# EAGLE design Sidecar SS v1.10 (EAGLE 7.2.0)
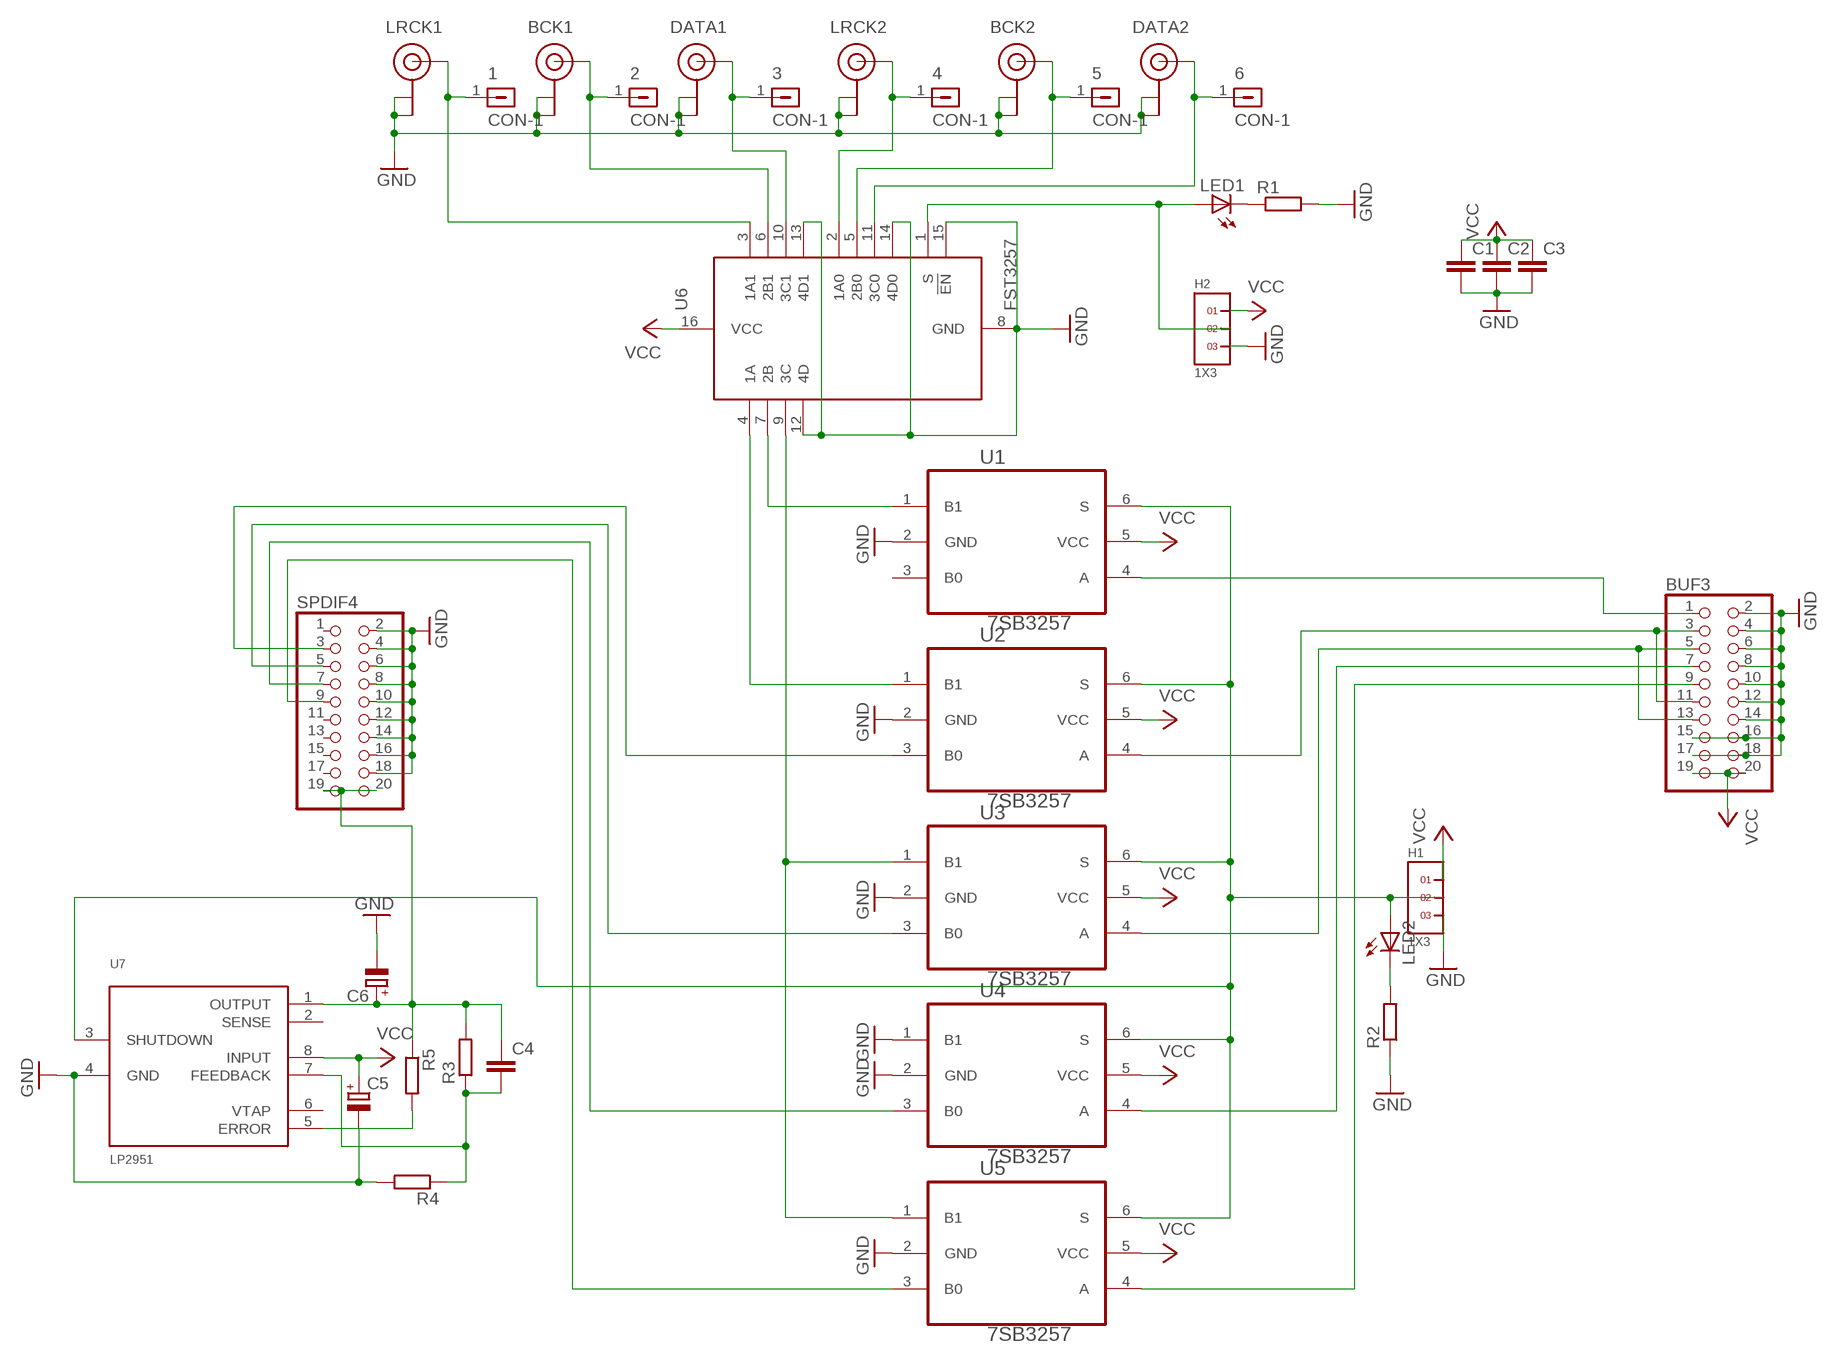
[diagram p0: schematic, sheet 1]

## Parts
1  CON-1  [CON-1]
2  CON-1  [CON-1]
3  CON-1  [CON-1]
4  CON-1  [CON-1]
5  CON-1  [CON-1]
6  CON-1  [CON-1]
BCK1  U.FL  [U.FL]
BCK2  U.FL  [U.FL]
BUF3  PINHD-2X10  [2X10]
C1  C-EUC0805  [C0805]
C2  C-EUC0805  [C0805]
C3  C-EUC0805  [C0805]
C4  C-EUC1206  [C1206]
C5  CPOL-EUCT3216  [CT3216]
C6  CPOL-EUCT3216  [CT3216]
DATA1  U.FL  [U.FL]
DATA2  U.FL  [U.FL]
H1  1X3  [1X3]
H2  1X3  [1X3]
LED1  LED_E  [LED_1206]
LED2  LED_E  [LED_1206]
LRCK1  U.FL  [U.FL]
LRCK2  U.FL  [U.FL]
R1  R-EU_R1206  [R1206]
R2  R-EU_R1206  [R1206]
R3  R-EU_R1206  [R1206]
R4  R-EU_R1206  [R1206]
R5  R-EU_R1206  [R1206]
SPDIF4  PINHD-2X10  [2X10]
U1  7SB3257  [TSOP-6]
U2  7SB3257  [TSOP-6]
U3  7SB3257  [TSOP-6]
U4  7SB3257  [TSOP-6]
U5  7SB3257  [TSOP-6]
U6  FST3257  [TSSOP16]
U7  LP2951  [SOIC-8]

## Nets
GND: BCK1.P$1(GND) BCK1.P$2(GND) BCK2.P$1(GND) BCK2.P$2(GND) BUF3.2 BUF3.4 BUF3.6 BUF3.8 BUF3.10 BUF3.12 BUF3.14 BUF3.15 BUF3.16 BUF3.17 BUF3.18 C1.2 C2.2 C3.2 C5.- C6.- DATA1.P$1(GND) DATA1.P$2(GND) DATA2.P$1(GND) DATA2.P$2(GND) H1.3 H2.3 LRCK1.P$1(GND) LRCK1.P$2(GND) LRCK2.P$1(GND) LRCK2.P$2(GND) R1.2 R2.1 R4.2 SPDIF4.2 SPDIF4.4 SPDIF4.6 SPDIF4.8 SPDIF4.10 SPDIF4.12 SPDIF4.14 SPDIF4.16 SPDIF4.18 U1.2(GND) U2.2(GND) U3.2(GND) U4.1(B1) U4.2(GND) U5.2(GND) U6.8(GND) U6.12(4D) U6.13(4D1) U6.14(4D0) U6.15(!EN) U7.4(GND)
N$1: C4.2 R3.1 R4.1 U7.7(FEEDBACK)
N$2: U1.1(B1) U6.7(2B)
N$3: SPDIF4.3 U2.3(B0)
N$4: BUF3.5 BUF3.13 U3.4(A)
N$5: BUF3.3 BUF3.11 U2.4(A)
N$6: BUF3.1 U1.4(A)
N$7: SPDIF4.5 U3.3(B0)
N$8: SPDIF4.7 U4.3(B0)
N$9: BUF3.7 U4.4(A)
N$10: BUF3.9 U5.4(A)
N$11: SPDIF4.9 U5.3(B0)
N$12: H1.2 LED2.A U1.6(S) U2.6(S) U3.6(S) U4.6(S) U5.6(S) U7.3(SHUTDOWN)
N$14: LED1.C R1.1
N$15: U2.1(B1) U6.4(1A)
N$16: U3.1(B1) U5.1(B1) U6.9(3C)
N$17: 1.1 LRCK1.P$3(SIGNAL) U6.3(1A1)
N$18: 2.1 BCK1.P$3(SIGNAL) U6.6(2B1)
N$19: 3.1 DATA1.P$3(SIGNAL) U6.10(3C1)
N$20: 4.1 LRCK2.P$3(SIGNAL) U6.2(1A0)
N$21: 5.1 BCK2.P$3(SIGNAL) U6.5(2B0)
N$22: 6.1 DATA2.P$3(SIGNAL) U6.11(3C0)
N$23: LED2.C R2.2
N$25: C4.1 C6.+ R3.2 R5.1 SPDIF4.19 SPDIF4.20 U7.1(OUTPUT)
N$27: R5.2 U7.5(ERROR)
N$29: H2.2 LED1.A U6.1(S)
VCC: BUF3.19 BUF3.20 C1.1 C2.1 C3.1 C5.+ H1.1 H2.1 U1.5(VCC) U2.5(VCC) U3.5(VCC) U4.5(VCC) U5.5(VCC) U6.16(VCC) U7.8(INPUT)
Unconnected: SPDIF4.1 SPDIF4.11 SPDIF4.13 SPDIF4.15 SPDIF4.17 U1.3(B0) U7.2(SENSE) U7.6(VTAP)

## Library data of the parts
1-6 = Dimdim:CON-1
BCK1 BCK2 DATA1 DATA2 LRCK1 LRCK2 = Dimdim:U.FL
BUF3 SPDIF4 = SparkFun-Connectors:PINHD-2X10: PIN HEADER
C1-C4 = rcl:C-EU: CAPACITOR, European symbol
C5 C6 = rcl:CPOL-EU: POLARIZED CAPACITOR, European symbol
H1 H2 = headers(.1in):1X3
LED1 LED2 = eagle-ltspice:LED_E: LED; SPICEMODEL: NONE; SPICEPREFIX: D; SPICETYPE: diode
R1-R5 = rcl:R-EU_: RESISTOR, European symbol
U1-U5 = Dimdim:7SB3257
U6 = Dimdim:FST3257
U7 = Dimdim:LP2951

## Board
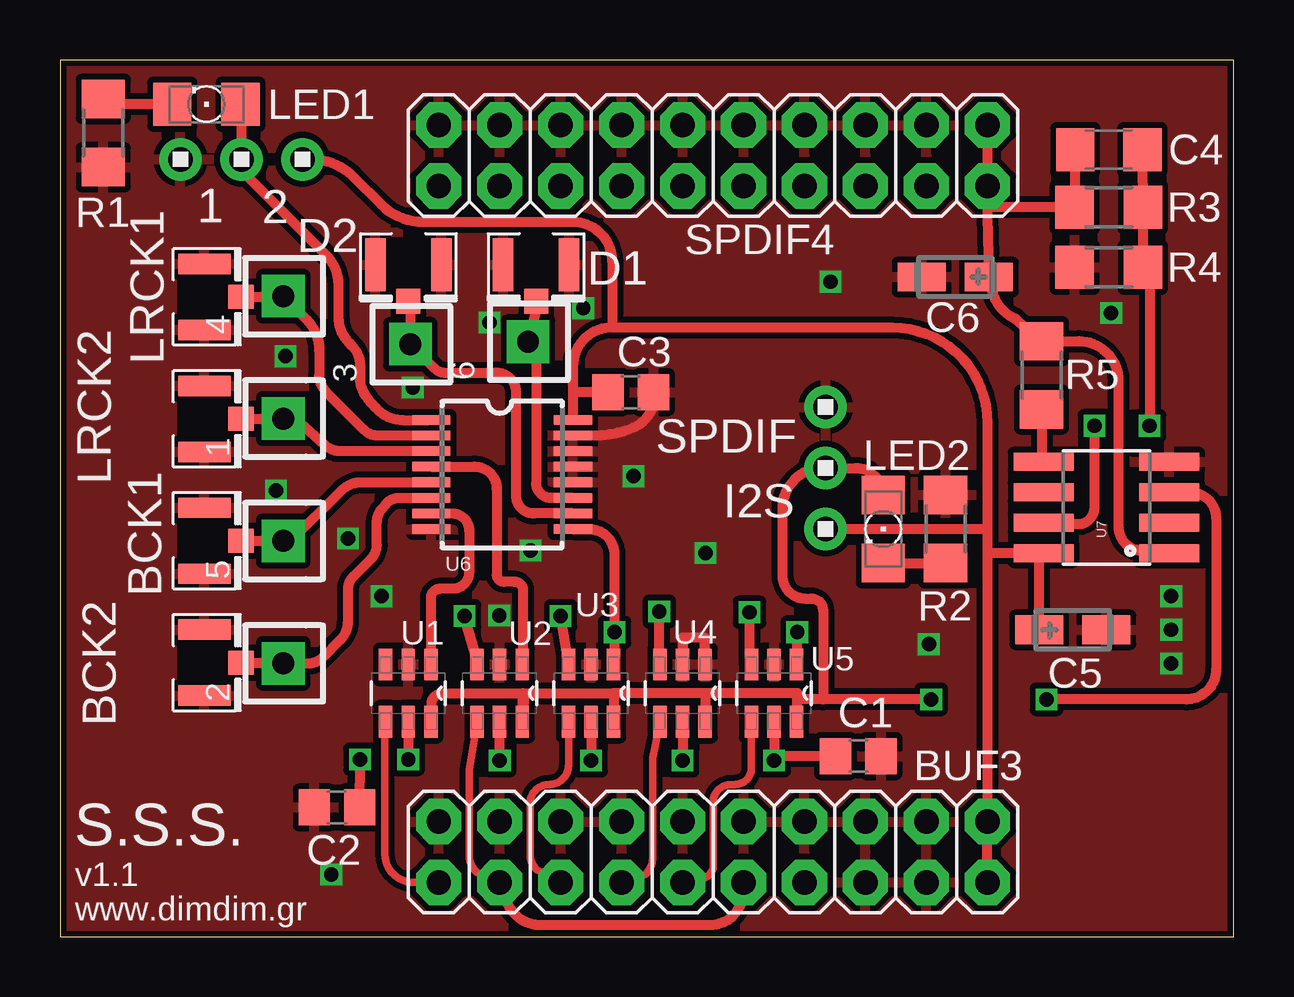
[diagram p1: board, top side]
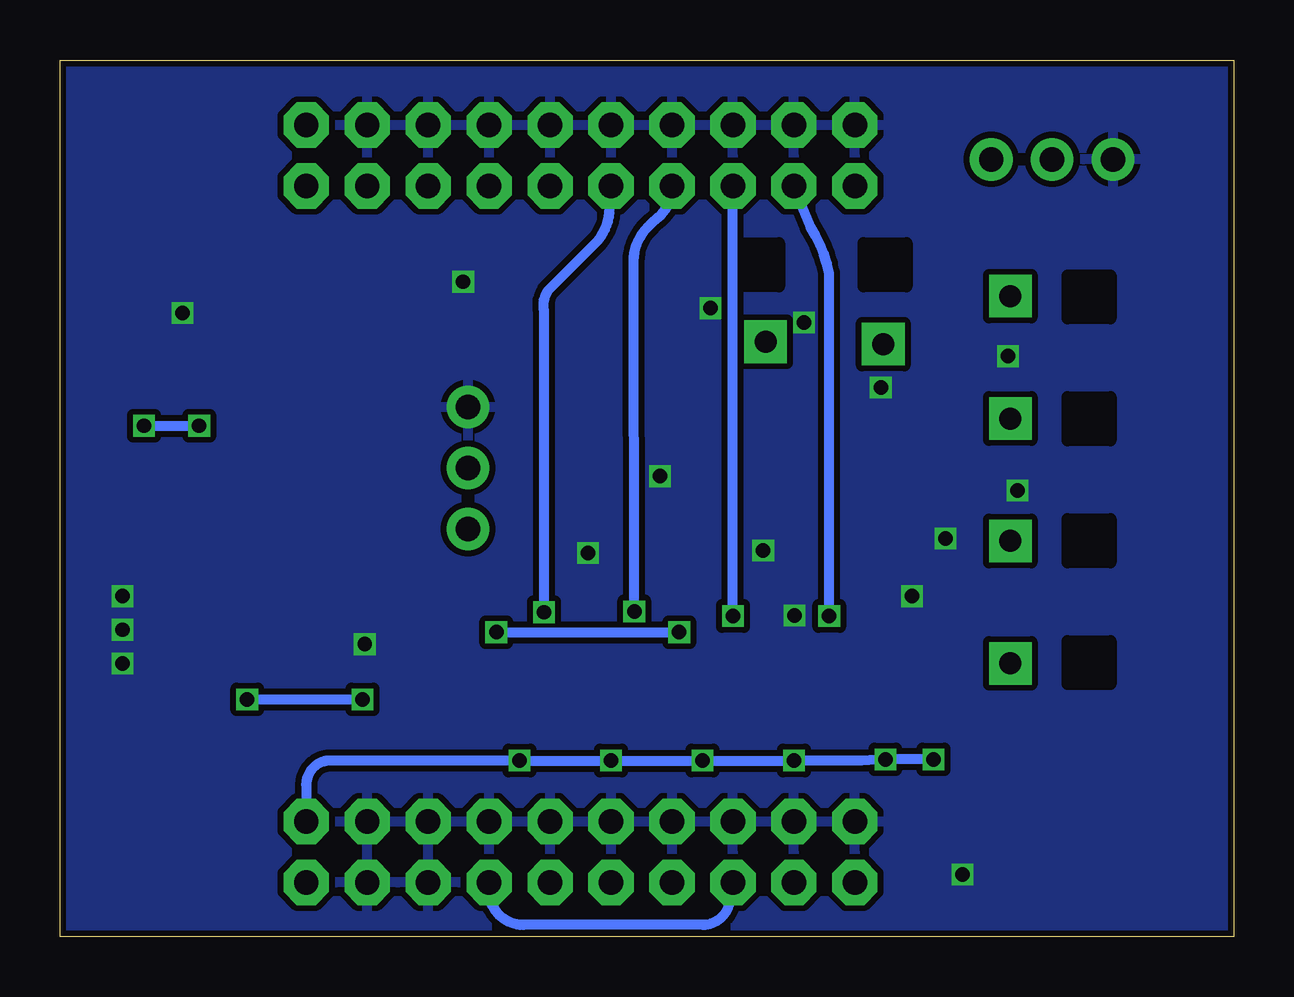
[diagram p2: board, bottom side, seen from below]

Size 48.9 x 36.54 mm. Coordinates in mm from the lower left corner, seen from the top.
Outline: 0,0 48.9,0 48.9,36.54 0,36.54 0,0
Copper layers (1*16): Top 0.035mm / dielectric 1.5mm / Bottom 0.035mm
Design rules "SeeedStudio_2layer_DRU_no_angle_20140221": minimum track width 6mil, minimum drill 12mil, track to track 6mil, track to pad 6mil, pad to pad 6mil, via to via 6mil, smd to smd 0mil, copper to edge 10mil, drill to drill 10mil, minimum pad ring 10mil, minimum via ring 6mil, stop-mask expansion 2mil, vias tented up to drill 100mil, thermal gap 10mil

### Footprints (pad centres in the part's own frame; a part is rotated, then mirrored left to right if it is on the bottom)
CON-1 = drill 0.914 pad 1.778 square: 1 0,0
U.FL = smd 2.2 x 0.85: P$1 0,1.375; P$2 0,-1.375 | smd 1.05 x 1: P$3 1.525,0
2X10 = drill 1.016 pad 1.88 octagon: 1 -11.43,-1.27; 2 -11.43,1.27; 3 -8.89,-1.27; 4 -8.89,1.27; 5 -6.35,-1.27; 6 -6.35,1.27; 7 -3.81,-1.27; 8 -3.81,1.27; 9 -1.27,-1.27; 10 -1.27,1.27; 11 1.27,-1.27; 12 1.27,1.27; 13 3.81,-1.27; 14 3.81,1.27; 15 6.35,-1.27; 16 6.35,1.27; 17 8.89,-1.27; 18 8.89,1.27; 19 11.43,-1.27; 20 11.43,1.27
C0805 = smd 1.3 x 1.5: 1 -0.95,0; 2 0.95,0
C1206 = smd 1.6 x 1.8: 1 -1.4,0; 2 1.4,0
CT3216 = smd 2 x 1.2: + -1.4,0; - 1.4,0
1X3 = drill 1.016 pad 1.778: 1 0,0; 2 2.54,0; 3 5.08,0
LED_1206 = smd 1.6 x 1.803: A -1.422,0; C 1.422,0
R1206 = smd 1.6 x 1.803: 1 -1.422,0; 2 1.422,0
TSOP-6 = smd 1.321 x 0.559: 1 -1.194,2.21; 2 -1.194,1.27; 3 -1.194,0.33; 4 1.194,0.33; 5 1.194,1.27; 6 1.194,2.21
TSSOP16 = smd 0.4 x 1.6: 1 -2.225,-2.85; 2 -1.575,-2.85; 3 -0.925,-2.85; 4 -0.275,-2.85; 5 0.375,-2.85; 6 1.025,-2.85; 7 1.675,-2.85; 8 2.325,-2.85; 9 2.325,3.05; 10 1.675,3.05; 11 1.025,3.05; 12 0.375,3.05; 13 -0.275,3.05; 14 -0.925,3.05; 15 -1.575,3.05; 16 -2.225,3.05
SOIC-8 = smd 0.75 x 2.5: 1 -1.905,-2.616; 2 -0.635,-2.616; 3 0.635,-2.616; 4 1.905,-2.616; 5 1.905,2.616; 6 0.635,2.616; 7 -0.635,2.616; 8 -1.905,2.616

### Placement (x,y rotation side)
1  9.3,21.6 0 top
2  9.3,11.4 0 top
3  14.6,24.7 0 top
4  9.3,26.7 0 top
5  9.3,16.5 0 top
6  19.5,24.8 0 top
BCK1  6.02,11.43 0 top
BCK2  6.02,16.51 0 top
BUF3  27.21,3.54 0 top
C1  33.26,7.54 0 top
C2  11.54,5.4 180 top
C3  23.78,22.7 0 top
C4  43.7,32.8 0 top
C5  42.2,12.8 0 top
C6  37.3,27.5 180 top
DATA1  14.52,28.01 270 top
DATA2  19.84,28.01 270 top
H1  31.9,17 90 top
H2  10.1,32.4 180 top
LED1  6.1,34.7 180 top
LED2  34.3,17 270 top
LRCK1  6.02,21.59 0 top
LRCK2  6.02,26.67 0 top
R1  1.8,33.5 270 top
R2  36.9,17 270 top
R3  43.7,30.4 180 top
R4  43.7,27.9 180 top
R5  40.9,23.4 270 top
SPDIF4  27.21,32.56 0 top
U1  13.24,10.16 270 top
U2  17.05,10.16 270 top
U3  20.86,10.16 270 top
U4  24.67,10.16 270 top
U5  28.48,10.16 270 top
U6  18.32,19.32 270 top
U7  43.6,17.9 90 top

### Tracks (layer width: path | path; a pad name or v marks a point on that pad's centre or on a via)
GND  (via drill 0.6)
  Top 0.406: U6.15 22.25,20.89 arc22 23.88,21.22 arc68 24.8,22.6 24.8,22.63 C3.2 | U4.1 26.86,11.35 26.86,12.47 25.94,12.47 U4.2
  other vias: 19.6,16.1 13.4,14.2 9.4,24.2 9,18.6 12,16.6 23.9,19.2 26.9,16 36.2,12.2 11.3,2.6 43.8,26 32.1,27.3 14.7,22.9 18.3,13.4 17.9,25.6 21.8,26.2 46.3,12.8 46.3,14.2 46.3,11.4
  pour Top (isolate 0.254): 0,36.6 48.92,36.6 48.92,0 0,0
  pour Bottom (isolate 0.254): 0,36.37 48.92,36.37 48.92,0 0,0
N$1  (via drill 0.6)
  Top 0.406: C4.2 45.1,32.42 R3.1 R4.1 | R4.1 45.2,28.4 | U7.7 40.98,17.2 42.43,17.2 arc59 42.99,17.52 arc31 43.1,17.92 v43.1,21.3 | R4.1 45.4,27.4 v45.4,21.3
  Bottom 0.406: v45.4,21.3 v43.1,21.3
N$2
  Top 0.406: U6.7 16.34,17.64 arc-90 17.05,16.94 17.05,15.2 arc-90 16.36,14.51 15.85,14.51 arc90 15.45,14.11 U1.1
N$3  (via drill 0.6)
  Top 0.406: U2.3 17.38,11.53 v16.85,13.37
  Bottom 0.406: v16.85,13.37 16.85,27.66 arc-22 17.62,29.57 SPDIF4.3
N$4
  Top 0.305: U3.4 21.19,7.16 arc-90 20.38,6.35 arc90 19.59,5.56 19.59,3.45 arc44 19.86,2.8 BUF3.5
  Bottom 0.406: BUF3.13 31.02,1.93 arc-90 29.59,0.5 22.12,0.5 arc-90 21,1.62 21,2.27 BUF3.5
N$5
  Top 0.305: U2.4 17.06,6.98 17.05,6.98 17.05,3.38 arc46 17.38,2.68 BUF3.3
  Top 0.406: BUF3.3 18.5,2.27 18.5,1.98 arc90 20.08,0.5 27.08,0.5 arc90 28.48,1.9 BUF3.11
N$6
  Top 0.305: 13.54,8.97 13.54,3.52 arc90 14.66,2.27 BUF3.1
  Top 0.406: U1.4 13.54,8.97
N$7  (via drill 0.6)
  Top 0.406: U3.3 v20.86,13.37
  Bottom 0.406: v20.86,13.37 SPDIF4.5 20.69,31.29
N$8  (via drill 0.6)
  Top 0.406: U4.3 24.97,11.45 v24.97,13.56
  Bottom 0.406: v24.97,13.56 25,28.13 arc49 24.29,29.7 23.95,30 arc-49 23.4,31.21 SPDIF4.7
N$9
  Top 0.305: U4.4 24.7,7.47 24.69,3.89 24.7,3.32 arc-50 24.36,2.58 BUF3.7
N$10
  Top 0.305: U5.4 28.81,7.04 arc-90 28.12,6.35 27.97,6.35 arc90 27.21,5.59 27.21,2.83 arc-52 26.77,2.42 BUF3.9
N$11  (via drill 0.6)
  Top 0.406: U5.3 28.74,11.32 v28.73,13.53
  Bottom 0.406: v28.73,13.53 28.73,26.1 arc45 28.56,26.94 26.6,28.9 arc-45 26,30.35 26,31.23 SPDIF4.9
N$12  (via drill 0.6)
  Top 0.406: U1.6 15.48,8.97 15.48,9.75 arc-90 15.97,10.15 19.34,10.15 | 19.29,10.16 19.34,10.15 | 19.34,10.15 U2.6 19.29,8.97 19.29,10.16 | 19.29,10.16 23.07,10.16 | 23.07,10.16 U3.6 | U4.6 26.91,8.97 26.91,10.16 | 26.91,10.16 23.07,10.16 | U5.6 30.72,8.97 30.72,9.9 | 30.72,9.9 30.72,10.1 | 26.91,10.16 30.72,10.16 30.72,10.1 | 31.8,9.9 31.8,13.6 arc90 31.3,14.1 31.05,14.1 arc-90 30.1,15.05 30.1,18.06 arc-90 32.08,19.54 H1.2 33.14,19.54 arc-88 LED2.A | 30.74,10.1 30.72,10.1 | v36.3,9.9 31.8,9.9 | 31.8,9.9 30.72,9.9 | U7.3 47.08,18.54 arc-90 48.17,17.45 48.17,11.14 arc-90 46.93,9.9 v41.1,9.9
  Bottom 0.406: v41.1,9.9 v36.3,9.9
N$14
  Top 0.406: LED1.C 1.32,34.7 R1.1
N$15
  Top 0.406: U6.4 17.28,19.59 arc-90 18.2,18.68 18.2,15.1 arc0 18.2,15.1 arc90 18.5,14.8 18.94,14.8 arc-90 19.3,14.44 19.3,11.55 19.29,11.55 U2.1
N$16  (via drill 0.6)
  Top 0.406: U6.9 22.04,17 arc-90 23.1,15.94 v23.1,12.7 23.1,11.73 23.07,11.43 U3.1 | U5.1 30.72,11.35 v30.72,12.7
  Bottom 0.406: v30.72,12.7 v23.1,12.7
N$17
  Top 0.406: LRCK1.P$3 1.1 9.8,21.6 11.01,20.51 arc42 11.69,20.25 15.41,20.25 U6.3
N$18
  Top 0.406: BCK1.P$3 9.27,11.43 2.1 10.36,11.4 arc45 10.94,11.64 11.7,12.4 arc45 12,13.13 12,14.5 arc-45 12.21,15.01 12.96,15.76 arc45 13.2,16.33 13.2,17.28 arc-41 13.41,17.84 13.58,18.05 arc-49 14.13,18.3 15.38,18.3 U6.6
N$19
  Top 0.406: U6.10 19.75,17.64 arc-90 19,18.4 19,22.8 arc90 18.1,23.5 16.08,23.5 arc-45 15.6,23.7 3.1 14.6,26.41 DATA1.P$3
N$20
  Top 0.406: U6.2 13.26,20.89 arc-45 12.66,21.14 11.08,22.72 arc-45 10.8,23.39 10.8,24.44 arc45 10.26,25.74 4.1 9.27,26.67 LRCK2.P$3
N$21
  Top 0.406: U6.5 12.55,18.95 arc45 11.73,18.6 9.62,16.5 5.1 BCK2.P$3
N$22
  Top 0.406: U6.11 20.46,18.3 arc-90 19.84,18.91 19.84,23.94 6.1 19.9,26.43 DATA2.P$3
N$23
  Top 0.406: LED2.C R2.2
N$25
  Top 0.406: SPDIF4.20 SPDIF4.19 | SPDIF4.19 38.64,30.06 C6.+ 38.8,27.27 arc68 39.81,25.77 R5.1 42.46,24.82 arc-90 44.1,23.18 44.1,17.1 arc90 45.1,16.1 46.22,16.1 U7.1 | C4.1 42.3,30.4 R3.2 38.64,30.4 SPDIF4.19
N$27
  Top 0.406: R5.2 40.9,19.89 U7.5
N$29
  Top 0.406: LED1.A 7.56,34.7 H2.2 7.56,31.94 11.08,28.42 arc-45 11.6,27.16 11.6,25.8 arc45 12.03,24.77 12.16,24.64 arc-45 12.5,23.82 12.5,23.27 arc41 12.81,22.45 13.16,22.05 arc49 14.29,21.54 15.32,21.54 U6.1
VCC  (via drill 0.6)
  Top 0.406: U1.5 v14.51,7.4 | v18.32,7.35 U2.5 | U3.5 v22.13,7.35 | U4.5 v25.94,7.35 | U5.5 v29.75,7.35 29.75,7.2 29.91,7.54 C1.1 | 23,25.4 arc90 21.37,23.77 21.37,22.7 | 23,25.4 34.67,25.4 arc-90 38.64,21.43 38.64,17 | 38.64,17 38.64,16.1 | 38.64,16.1 BUF3.20 BUF3.19 38.64,2.58 | C2.1 v12.5,7.4 | H1.1 38.64,17 | 23,25.4 23,28.16 arc90 21.36,29.8 15.12,29.8 arc-45 13.38,30.52 12.2,31.7 arc45 10.5,32.4 H2.1 | 38.64,16.1 38.74,15.99 U7.8 40.8,15.81 C5.+ | C3.1 21.37,22.7 | 21.37,22.7 U6.16
  Bottom 0.406: BUF3.20 38.64,6.34 arc90 37.63,7.35 v29.75,7.35 v25.94,7.35 v22.13,7.35 v18.32,7.35 15.51,7.35 v14.51,7.4 v12.5,7.4

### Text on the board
tNames: 1 | 2 | LRCK1 | D2 | D1 | LRCK2 | SPDIF | BCK1 | I2S | BCK2 | S.S.S. | v1.1 | www.dimdim.gr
